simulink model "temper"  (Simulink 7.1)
settings: Solver=ode45  StartTime=0.0  StopTime=20  MaxStep=0.1  RelTol=1e-3  AbsTol=1e-3

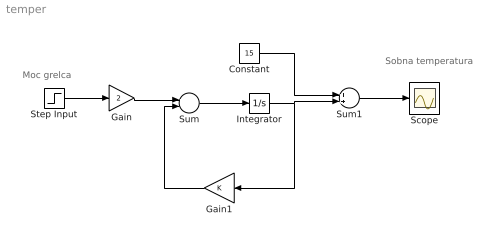
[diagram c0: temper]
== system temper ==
  note: Moc grelca
  note: Sobna temperatura
  Constant : Constant  Value=15
  Gain : Gain  Gain=2
  Gain1 : Gain  Orientation=left
  Integrator : Integrator
  Scope : Scope
  Step Input : Step  Time=0  After=5  SampleTime=0
  Sum : Sum  Inputs=+-
  Sum1 : Sum
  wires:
  Step Input/1 -> Gain/1
  Gain/1 -> Sum/1
  Sum/1 -> Integrator/1
  Gain1/1 -> Sum/2
  Integrator/1 -> Gain1/1, Sum1/2
  Constant/1 -> Sum1/1
  Sum1/1 -> Scope/1
